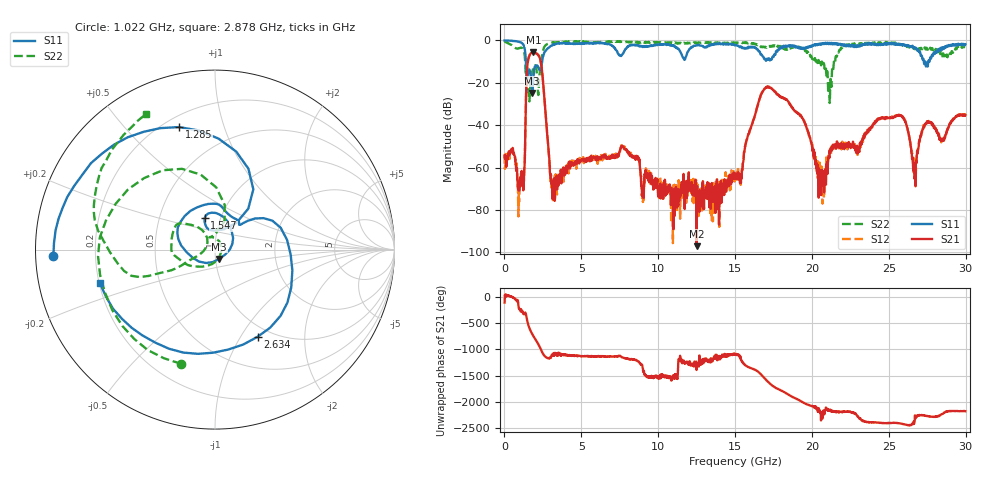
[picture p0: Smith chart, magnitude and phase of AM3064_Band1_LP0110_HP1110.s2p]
# Hz S DB R 50.0
!freq dBS11 angS11 dBS21 angS21 dBS12 angS12 dBS22 angS22
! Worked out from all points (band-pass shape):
!   1600 points, 10 MHz to 29.98 GHz, reference 50 ohm
!   highest |S21| = -5.66 dB at 1.884 GHz (marker M1); lowest = -97.1 dB at 12.49 GHz (marker M2)
!   |S21| within 3 dB of the highest: 1.558 GHz to 2.309 GHz (750.8 MHz wide, 38.8 % of centre)
!   lowest |S11| = -24.8 dB at 1.809 GHz (marker M3), VSWR 1.12, Z = 52.1 - j5.5 ohm
!   |S11| at or under -10 dB: 1.393 GHz to 2.444 GHz (1.051 GHz wide, 54.8 % of centre); 27.28234 GHz to 27.3521 GHz (69.76 MHz wide, 0.255 % of centre); 27.36 GHz to 27.57 GHz (209.2 MHz wide, 0.762 % of centre)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
!   |S22| runs from -29.6 to -0.4 dB; largest |S21 - S12| = 0.0082
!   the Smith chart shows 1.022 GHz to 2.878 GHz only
!   S11 on the Smith chart (normalised r, x): 1.022 GHz: 0.05, -0.02; 1.285 GHz: 0.26, +0.72; 1.547 GHz: 0.84, +0.30; 2.634 GHz: 0.86, -1.19; 2.878 GHz: 0.20, -0.14
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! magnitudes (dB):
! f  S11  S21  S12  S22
! 10 MHz  -0.1  -54.3  -54.1  -0.4
! 1.022 GHz  -0.9  -65.2  -66.1  -3.6
! 1.285 GHz  -3.0  -61.2  -63.0  -5.5
! 1.547 GHz  -14.7  -9.0  -8.9  -22.9
! 1.809 GHz  -24.8  -5.8  -5.7  -14.7
! 1.884 GHz  -17.6  -5.7  -5.7  -12.8
! 2.634 GHz  -5.3  -30.8  -30.7  -2.7
! 2.878 GHz  -3.5  -53.0  -53.0  -1.5
! 3.159 GHz  -2.2  -73.5  -76.1  -1.1
! 5.015 GHz  -1.4  -56.6  -56.9  -0.7
! 7.714 GHz  -6.3  -50.1  -49.6  -0.7
! 10 GHz  -2.0  -73.7  -69.2  -0.9
! 12.49 GHz  -2.3  -97.1  -67.4  -1.1
! 15 GHz  -2.2  -63.6  -65.2  -1.3
! 17.05 GHz  -9.1  -22.0  -22.1  -3.5
! 19.99 GHz  -3.0  -49.5  -48.7  -8.2
! 20.67 GHz  -1.6  -68.2  -63.7  -10.3
! 25 GHz  -1.3  -36.6  -36.5  -1.2
! 26.01 GHz  -2.5  -37.2  -37.2  -2.1
! 26.66 GHz  -3.2  -62.2  -60.0  -3.9
! 27.41 GHz  -12.4  -39.1  -38.7  -4.3
! 29.98 GHz  -1.8  -35.3  -35.4  -2.8
